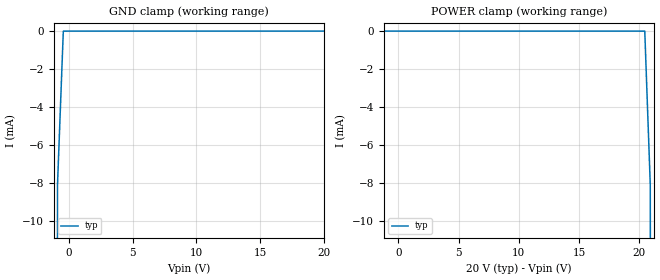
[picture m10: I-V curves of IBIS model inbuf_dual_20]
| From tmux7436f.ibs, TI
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| inbuf_dual_20
[Model]   inbuf_dual_20
Model_type   Input
Vinl = 0.8
Vinh = 1.3
|   typ   min   max
C_comp   6.362683e-13   NA   NA
[Voltage Range]   20   NA   NA
[Temperature Range]   27   NA   NA
[Power Clamp Reference]   20   NA   NA
[GND Clamp Reference]   0   NA   NA
[GND Clamp]
|   Voltage   I(typ)   I(min)   I(max)
-25V      -12.14A    NA         NA
-1.364V   -160.3mA   NA         NA
-909.1mV  -8.044mA   NA         NA
-454.5mV  -3.86uA    NA         NA
20V       1.246uA    NA         NA
[POWER Clamp]
|   Voltage   I(typ)   I(min)   I(max)
-5V       1.552uA    NA         NA
20.45V    -3.86uA    NA         NA
20.91V    -8.044mA   NA         NA
21.36V    -160.3mA   NA         NA
40V       -9.607A    NA         NA
